(* Logix 5000 Routine export RTA_SCNDR; software revision 32.00 *)

TYPE RTA_SCNDR_Dual_Scanner :
STRUCT
   Heartbeat : INT;   // Controller scope tag that the 435NBX updates with a free running counter to let the PLC know the 435NBX is present and actively communicating.
   Active : BOOL;   // Controller scope tag that the RTA_SCNDR_Heartbeat AOI uses to let the PLC show an active connection.
   P0_Received_Garbage_Data : BOOL;   // Controller scope tag that the RTA_SCNDR_P0_Barcode_Scanner_to_PLC AOI uses to indicate that it received data that was garbage. Potentially due to removal of cable to scanner or removal of power from the scanner.
   P1_Received_Garbage_Data : BOOL;   // Controller scope tag that the RTA_SCNDR_P1_Barcode_Scanner_to_PLC AOI uses to indicate that it received data that was garbage. Potentially due to removal of cable to scanner or removal of power from the scanner.
   P0_ASCII_Data : RTA_STRING_4096;   // Controller scope tag that the RTA 435NBX writes the ASCII data received from the barcode scanner on port 0 to the RTA_SCNDR_P0_Barcode_Scanner_to_PLC AOI
   P0_Barcode_Data : RTA_STRING_4096;   // Controller scope tag that the RTA_SCNDR_P0_Barcode_Scanner_to_PLC AOI uses to make data available to the PLC program.
   P1_ASCII_Data : RTA_STRING_4096;   // Controller scope tag that the RTA 435NBX writes the ASCII data received from the barcode scanner on port 1 to the RTA_SCNDR_P1_Barcode_Scanner_to_PLC AOI
   P1_Barcode_Data : RTA_STRING_4096;   // Controller scope tag that the RTA_SCNDR_P1_Barcode_Scanner_to_PLC AOI uses to make data available to the PLC program.
END_STRUCT
END_TYPE

TYPE RTA_STRING_4096 :   // string type; String data type with up to 4096 characters available.
STRUCT
   LEN : DINT;
   DATA : SINT[4096];
END_STRUCT
END_TYPE

ADD_ON_INSTRUCTION RTA_SCNDR_Heartbeat_AOI   (* revision 1.0, vendor Real Time Automation, Inc. *)
// RTA's 435NBX heartbeat handshaking
VAR_IN_OUT
   DataIn : INT; {required}
   DataOut : BOOL; {required}
END_VAR
VAR
   Previous_Value : INT; {access None}
   Number_of_Times_Inactive : INT; {access None}
END_VAR

ROUTINE Logic   (* ladder *)
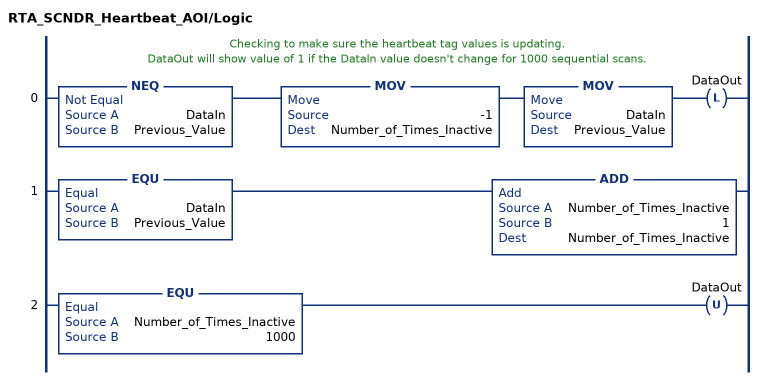
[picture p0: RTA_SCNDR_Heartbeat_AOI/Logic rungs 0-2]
   // Checking to make sure the heartbeat tag values is updating.
   // DataOut will show value of 1 if the DataIn value doesn't change for 1000 sequential scans.
   0: NEQ(DataIn,Previous_Value)MOV(-1,Number_of_Times_Inactive)MOV(DataIn,Previous_Value)OTL(DataOut);
   1: EQU(DataIn,Previous_Value)ADD(Number_of_Times_Inactive,1,Number_of_Times_Inactive);
   2: EQU(Number_of_Times_Inactive,1000)OTU(DataOut);
END_ROUTINE
END_ADD_ON_INSTRUCTION

ADD_ON_INSTRUCTION RTA_SCNDR_P0_Barcode_Scanner_to_PLC_AOI   (* revision 1.0, vendor Real Time Automation, Inc. *)
// RTA's 435NBX gateway to PLC handshaking
VAR_IN_OUT
   DataIn : RTA_STRING_4096; {required}
   DataOut : RTA_STRING_4096; {required}
   GarbageData : BOOL; {required}   // The Barcode Scanner is unplugged / unpowered
END_VAR
VAR
   CR_Offset : DINT; {access None}
   LF_Offset : DINT; {access None}
   LF : RTA_STRING_4096 := '$l'; {access None}
   CR : RTA_STRING_4096 := '$r'; {access None}
END_VAR

ROUTINE Logic   (* ladder *)
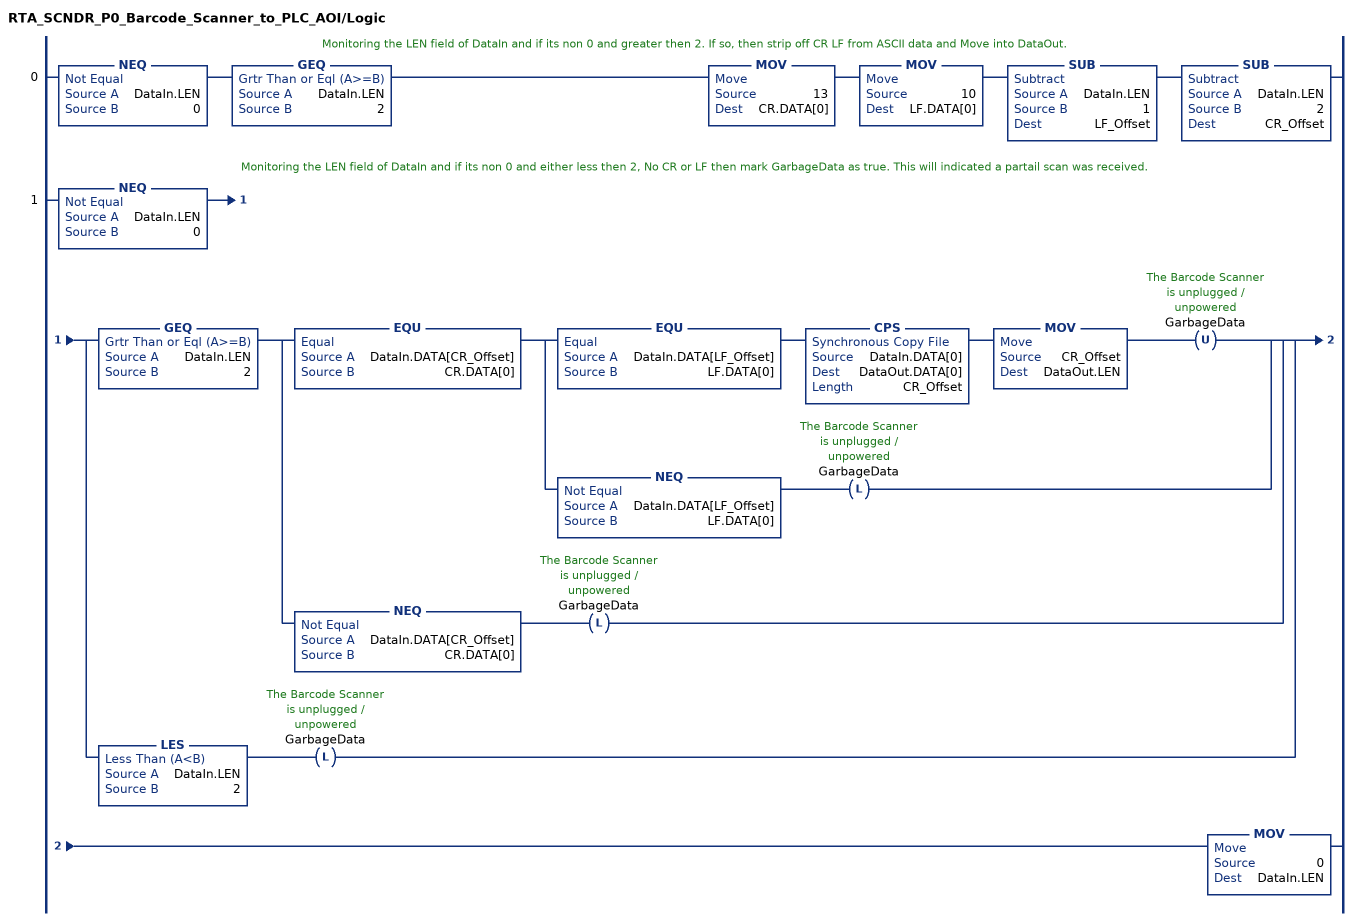
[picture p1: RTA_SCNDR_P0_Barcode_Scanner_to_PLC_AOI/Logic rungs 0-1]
   // Monitoring the LEN field of DataIn and if its non 0 and greater then 2. If so, then strip off CR LF from ASCII data and Move into DataOut.
   0: NEQ(DataIn.LEN,0)GEQ(DataIn.LEN,2)MOV(13,CR.DATA[0])MOV(10,LF.DATA[0])SUB(DataIn.LEN,1,LF_Offset)SUB(DataIn.LEN,2,CR_Offset);
   // Monitoring the LEN field of DataIn and if its non 0 and either less then 2, No CR or LF then mark GarbageData as true. This will indicated a partail scan was received.
   1: NEQ(DataIn.LEN,0)[GEQ(DataIn.LEN,2) [EQU(DataIn.DATA[CR_Offset],CR.DATA[0]) [EQU(DataIn.DATA[LF_Offset],LF.DATA[0]) CPS(DataIn.DATA[0],DataOut.DATA[0],CR_Offset) MOV(CR_Offset,DataOut.LEN) OTU(GarbageData) ,NEQ(DataIn.DATA[LF_Offset],LF.DATA[0]) OTL(GarbageData) ] ,NEQ(DataIn.DATA[CR_Offset],CR.DATA[0]) OTL(GarbageData) ] ,LES(DataIn.LEN,2) OTL(GarbageData) ]MOV(0,DataIn.LEN);
END_ROUTINE
END_ADD_ON_INSTRUCTION

ADD_ON_INSTRUCTION RTA_SCNDR_P1_Barcode_Scanner_to_PLC_AOI   (* revision 1.0, vendor Real Time Automation, Inc. *)
// RTA's 435NBX gateway to PLC handshaking
VAR_IN_OUT
   DataIn : RTA_STRING_4096; {required}
   DataOut : RTA_STRING_4096; {required}
   GarbageData : BOOL; {required}   // The Barcode Scanner is unplugged / unpowered
END_VAR
VAR
   CR_Offset : DINT; {access None}
   LF_Offset : DINT; {access None}
   LF : RTA_STRING_4096 := '$l'; {access None}
   CR : RTA_STRING_4096 := '$r'; {access None}
END_VAR

ROUTINE Logic   (* ladder *)
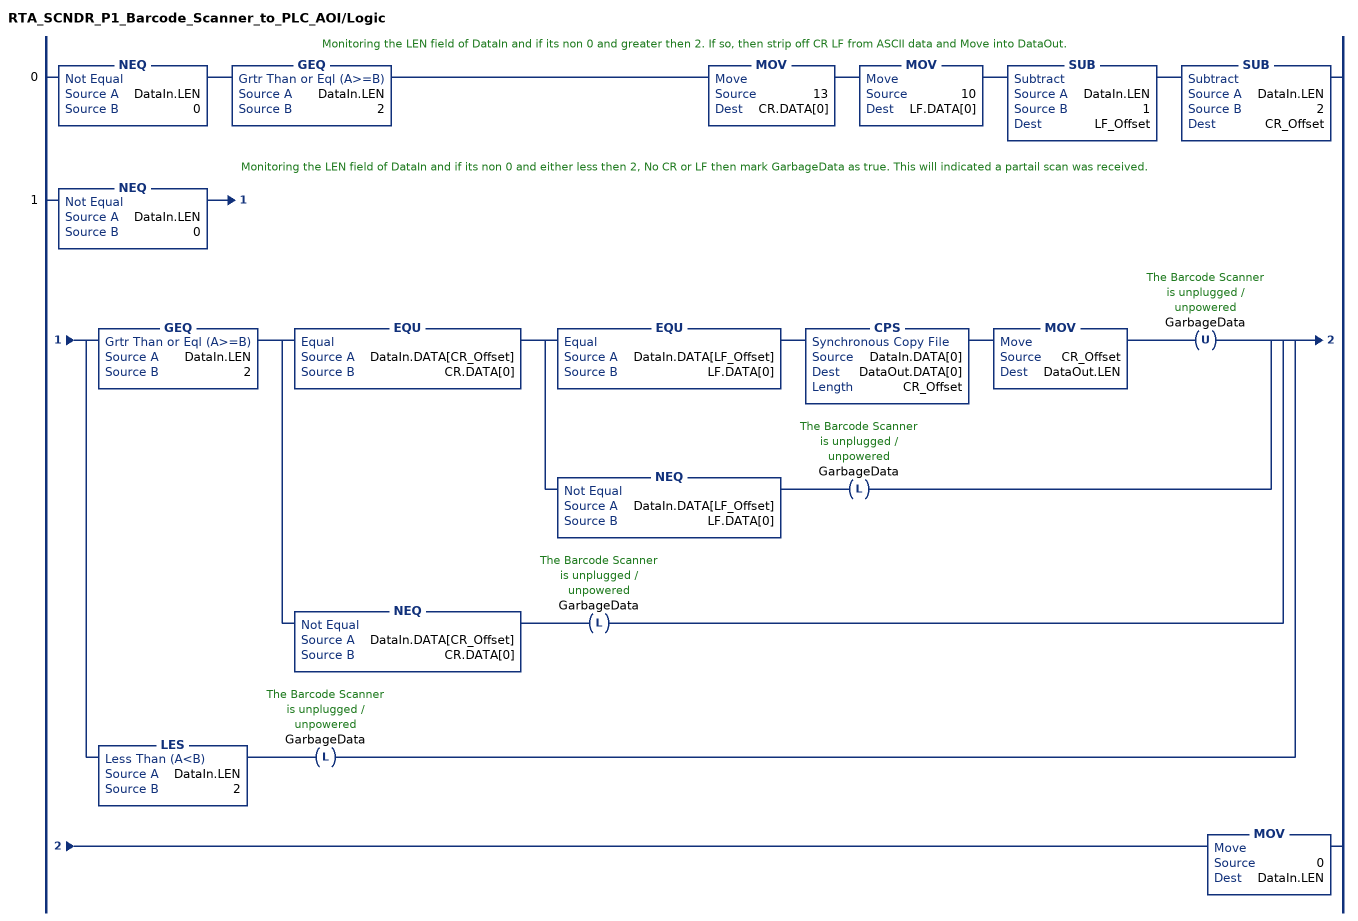
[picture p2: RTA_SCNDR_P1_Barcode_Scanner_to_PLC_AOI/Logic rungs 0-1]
   // Monitoring the LEN field of DataIn and if its non 0 and greater then 2. If so, then strip off CR LF from ASCII data and Move into DataOut.
   0: NEQ(DataIn.LEN,0)GEQ(DataIn.LEN,2)MOV(13,CR.DATA[0])MOV(10,LF.DATA[0])SUB(DataIn.LEN,1,LF_Offset)SUB(DataIn.LEN,2,CR_Offset);
   // Monitoring the LEN field of DataIn and if its non 0 and either less then 2, No CR or LF then mark GarbageData as true. This will indicated a partail scan was received.
   1: NEQ(DataIn.LEN,0)[GEQ(DataIn.LEN,2) [EQU(DataIn.DATA[CR_Offset],CR.DATA[0]) [EQU(DataIn.DATA[LF_Offset],LF.DATA[0]) CPS(DataIn.DATA[0],DataOut.DATA[0],CR_Offset) MOV(CR_Offset,DataOut.LEN) OTU(GarbageData) ,NEQ(DataIn.DATA[LF_Offset],LF.DATA[0]) OTL(GarbageData) ] ,NEQ(DataIn.DATA[CR_Offset],CR.DATA[0]) OTL(GarbageData) ] ,LES(DataIn.LEN,2) OTL(GarbageData) ]MOV(0,DataIn.LEN);
END_ROUTINE
END_ADD_ON_INSTRUCTION

VAR_GLOBAL   (* controller tags *)
   RTA_SCNDR_Heartbeat_AOI : RTA_SCNDR_Heartbeat_AOI;
   RTA_SCNDR_P0_AOI : RTA_SCNDR_P0_Barcode_Scanner_to_PLC_AOI;
   RTA_SCNDR_P1_AOI : RTA_SCNDR_P1_Barcode_Scanner_to_PLC_AOI;
   RTA_SCNDR_Tags : RTA_SCNDR_Dual_Scanner;
END_VAR

PROGRAM MainProgram

ROUTINE RTA_SCNDR   (* ladder *)
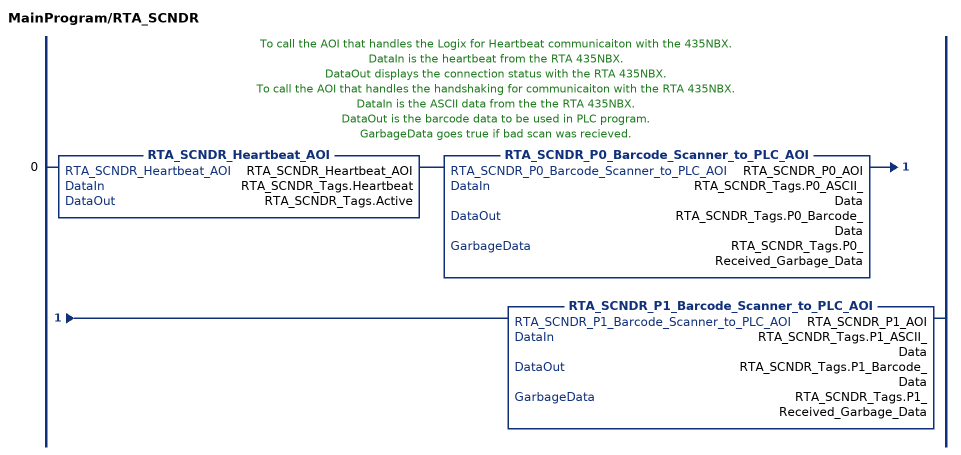
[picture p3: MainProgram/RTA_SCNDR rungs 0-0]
   // To call the AOI that handles the Logix for Heartbeat communicaiton with the 435NBX.
   // DataIn is the heartbeat from the RTA 435NBX.
   // DataOut displays the connection status with the RTA 435NBX.
   // To call the AOI that handles the handshaking for communicaiton with the RTA 435NBX.
   // DataIn is the ASCII data from the the RTA 435NBX.
   // DataOut is the barcode data to be used in PLC program.
   // GarbageData goes true if bad scan was recieved.
   0: RTA_SCNDR_Heartbeat_AOI(RTA_SCNDR_Heartbeat_AOI,RTA_SCNDR_Tags.Heartbeat,RTA_SCNDR_Tags.Active)RTA_SCNDR_P0_Barcode_Scanner_to_PLC_AOI(RTA_SCNDR_P0_AOI,RTA_SCNDR_Tags.P0_ASCII_Data,RTA_SCNDR_Tags.P0_Barcode_Data,RTA_SCNDR_Tags.P0_Received_Garbage_Data)RTA_SCNDR_P1_Barcode_Scanner_to_PLC_AOI(RTA_SCNDR_P1_AOI,RTA_SCNDR_Tags.P1_ASCII_Data,RTA_SCNDR_Tags.P1_Barcode_Data,RTA_SCNDR_Tags.P1_Received_Garbage_Data);
END_ROUTINE
END_PROGRAM
